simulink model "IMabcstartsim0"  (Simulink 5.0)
settings: Solver=ode45  StartTime=0.0  StopTime=4  MaxStep=1e-3  RelTol=1e-3
InitFcn:
  | imparamstartsim0
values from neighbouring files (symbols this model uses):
  Bm = 0.10    (= 0.1)    [IMabc2.m]    (also in imabcparam.m = 0.01; IMabcrun0.m = 0.01; IMabcrun1.m = 0.001; IMcur0.m = 1e-06)
  gam = 2*pi/3    (= 2.09439510239)    [IMabc2.m]    (also in IMabcf0.m; IMabcf1.m; imabcparam.m; IMabcrun0.m)
  H = 0.60    (= 0.6)    [IMabc2.m]    (also in IMcur0.m = 0.3; imdef0vec.m = 0.3; imdef1vec.m = 0.3; imdef2vec.m = 0.3)
  Lm1 = 2/3*Lm    [IMabcf0.m]    (also in IMabcf1.m; imabcparam.m = 0.0564666666667; IMabcrun0.m = 0.0564666666667; IMabcrun1.m = 0.0564666666667)
  Lr = Lrl+Lm    (= 4.6)    [IMabc2.m]    (also in IMabcf0.m = Lrl+Lm1; IMabcf1.m = Lrl+Lm1; imabcparam.m = 0.0589666666667; IMcur0.m)
  Ls = Lsl+Lm    (= 4.6)    [IMabc2.m]    (also in IMabcf0.m = Lsl+Lm1; IMabcf1.m = Lsl+Lm1; imabcparam.m = 0.0589666666667; IMcur0.m)
  Rr = input('Rotor resistance)[default = 2] =')    [Actac.m]    (also in im1phase.m = 0.3; im3d.m = eval(get(hRr,'String')); IMabc2.m = 0.02; imabcparam.m = 0.408)
  Rs = eval(get(hRs,'String'))    [im3d.m]    (also in IMabc2.m = 0.01; imabcparam.m = 0.531; IMabcrun0.m = 0.531; IMabcrun1.m = 0.531)
  Vm = Vll*sqrt(2/3)    [imabcparam.m]
  wo = 2*pi*freq0    [calc0.m]    (also in IMabc2.m = 376.991118431; imabcparam.m = 376.991118431; IMabcrun0.m = 376.991118431; IMabcrun1.m = 376.991118431)
undefined symbols (not defined in the file or in its folder): TL1, TL2
libraries: simulink x9

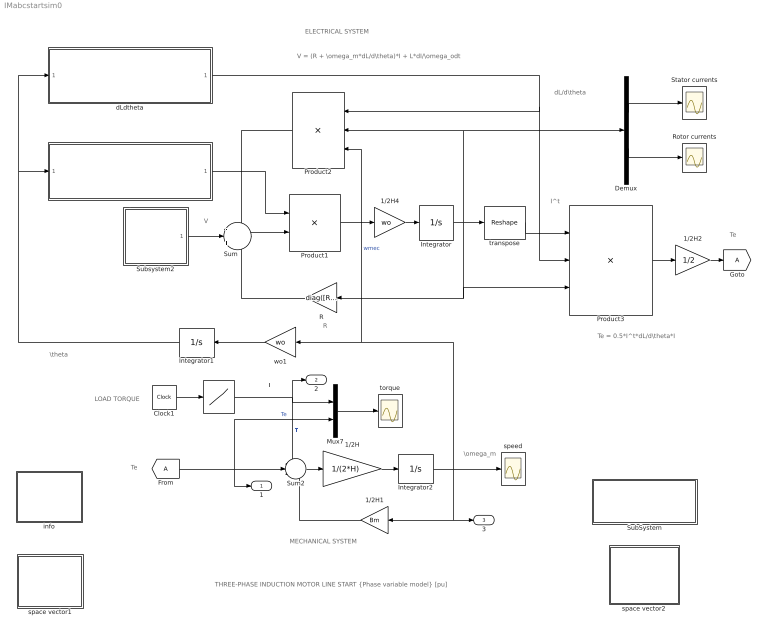
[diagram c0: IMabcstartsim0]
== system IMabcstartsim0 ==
  note: I
  note: I^t
  note: MECHANICAL SYSTEM
  note: ELECTRICAL SYSTEM
  note: V
  note: \omega_m
  note: \theta
  note: THREE-PHASE INDUCTION MOTOR LINE START {Phase variable model} [pu]
  note: L
  note: Te
  note: TL
  note: Te
  note: LOAD TORQUE
  note: R
  note: Te = 0.5*I^t*dL/d\theta*I
  note: V = (R + \omega_m*dL/d\theta)*I + L*dI/\omega_odt
  note: dL/d\theta
  " " : Lookup  InputValues="[0 2 2  4]"  OutputValues="[TL1 TL1  TL2  TL2]"
  1/2H : Gain  Gain=1/(2*H)
  1/2H1 : Gain  Orientation=left  Gain=Bm
  1/2H2 : Gain  Gain=1/2
  1/2H4 : Gain  Gain=wo
  Clock1 : Clock
  Demux : Demux  Outputs=2
  Integrator : Integrator  InitialCondition=[0 ;0 ;0; 0 ;0 ;0]
  Integrator1 : Integrator  Orientation=left
  Integrator2 : Integrator
  L : Subsystem
  Mux7 : Mux  Inputs=2
  Product1 : Product  Inputs=/*  Multiplication=Matrix(*)
  Product2 : Product  Orientation=left  Inputs=***  Multiplication=Matrix(*)
  Product3 : Product  Inputs=3  Multiplication=Matrix(*)  ShowAdditionalParam=on
  R : Gain  Orientation=left  Gain=diag([Rs Rs Rs Rr Rr Rr])  Multiplication=Matrix(K*u)
  Rotor currents : Scope
  Stator currents : Scope
  SubSystem : Subsystem
  Subsystem2 : Subsystem
  Sum : Sum  Inputs=-|+|-
  Sum2 : Sum  Inputs=-+-
  dLdtheta : Subsystem
  info : Subsystem
  space vector1 : Subsystem
  space vector2 : Subsystem
  speed : Scope
  torque : Scope
  transpose : simulink/Math Operations/Reshape  OutputDimensionality=Row vector  OutputDimensions=[1,6]
  wo1 : Gain  Orientation=left  Gain=wo
  1 : Outport
  2 : Outport  Port=2
  3 : Outport  Port=3
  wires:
  Product1/1 -> 1/2H4/1
  Sum/1 -> Product1/2
  R/1 -> Sum/3
  transpose/1 -> Product3/1
  Demux/1 -> Stator currents/1
  Demux/2 -> Rotor currents/1
  Product2/1 -> Sum/1
  dLdtheta/1(dLdtheta) -> Product2/1, Product3/2
  Product3/1 -> 1/2H2/1
  Sum2/1 -> 1/2H/1
  1/2H/1 -> Integrator2/1
  1/2H1/1 -> Sum2/3
  Mux7/1 -> torque/1
  " "/1 -> Mux7/1, Sum2/1, 2/1  "TL"
  [A] -> Sum2/2, 1/1, Mux7/2  "Te"
  Integrator2/1 -> Product2/3, wo1/1, speed/1, 1/2H1/1, 3/1  "wmec"
  Subsystem2/1(V) -> Sum/2
  Integrator1/1 -> dLdtheta/1(theta1), L/1(theta)
  L/1(L) -> Product1/1
  Clock1/1 -> " "/1
  1/2H2/1 -> [A]
  Integrator/1 -> transpose/1, Product2/2, Demux/1, R/1, Product3/3
  wo1/1 -> Integrator1/1
  1/2H4/1 -> Integrator/1

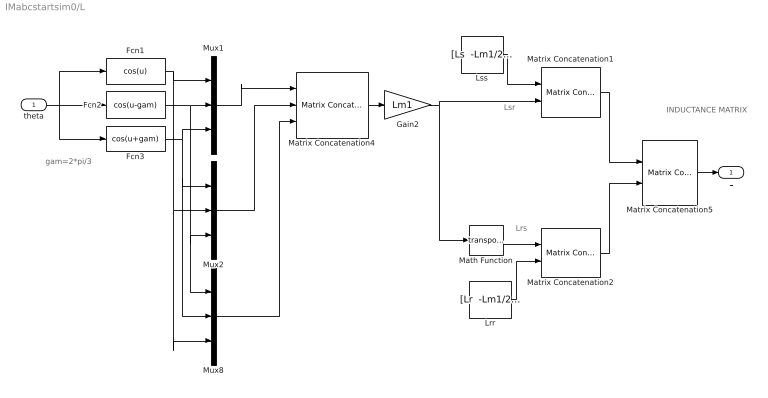
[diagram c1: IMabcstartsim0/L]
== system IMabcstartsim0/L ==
  note: Lrs
  note: Lsr
  note: INDUCTANCE MATRIX
  note: gam=2*pi/3
  theta : Inport
  Fcn1 : Fcn  Expr=cos(u)
  Fcn2 : Fcn  Expr=cos(u-gam)
  Fcn3 : Fcn  Expr=cos(u+gam)
  Gain2 : Gain  Gain=Lm1
  Lrr : Constant  Value="[Lr  -Lm1/2  -Lm1/2; -Lm1/2  Lr -Lm1/2;-Lm1/2  -Lm1/2  Lr]"  VectorParams1D=off
  Lss : Constant  Value="[Ls  -Lm1/2  -Lm1/2; -Lm1/2  Ls  -Lm1/2;-Lm1/2  -Lm1/2  Ls]"  VectorParams1D=off
  Math Function : Math  Operator=transpose
  Matrix Concatenation1 : simulink/Math Operations/Matrix Concatenation  numInports=2  catMethod=Horizontal
  Matrix Concatenation2 : simulink/Math Operations/Matrix Concatenation  numInports=2  catMethod=Horizontal
  Matrix Concatenation4 : simulink/Math Operations/Matrix Concatenation  numInports=3  catMethod=Horizontal
  Matrix Concatenation5 : simulink/Math Operations/Matrix Concatenation  numInports=2  catMethod=Vertical
  Mux1 : Mux  Inputs=3
  Mux2 : Mux  Inputs=3
  Mux8 : Mux  Inputs=3
  L : Outport
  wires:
  Fcn1/1 -> Mux1/1, Mux2/2, Mux8/3
  Fcn2/1 -> Mux8/1, Mux2/3, Mux1/2
  Fcn3/1 -> Mux8/2, Mux2/1, Mux1/3
  Lrr/1 -> Matrix Concatenation2/2
  Lss/1 -> Matrix Concatenation1/1
  Matrix Concatenation2/1 -> Matrix Concatenation5/2
  Matrix Concatenation1/1 -> Matrix Concatenation5/1
  Mux2/1 -> Matrix Concatenation4/2
  Mux8/1 -> Matrix Concatenation4/3
  Matrix Concatenation4/1 -> Gain2/1
  Mux1/1 -> Matrix Concatenation4/1
  Gain2/1 -> Math Function/1, Matrix Concatenation1/2
  Math Function/1 -> Matrix Concatenation2/1
  theta/1 -> Fcn2/1, Fcn1/1, Fcn3/1
  Matrix Concatenation5/1 -> L/1

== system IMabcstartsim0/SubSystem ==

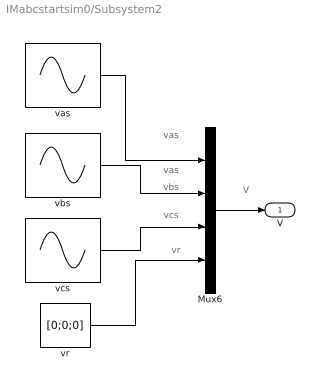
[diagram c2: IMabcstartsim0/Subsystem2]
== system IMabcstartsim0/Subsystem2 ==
  note: vas
  note: vas
  note: vbs
  note: vcs
  note: vr
  note: V
  Mux6 : Mux
  vas : Sin  Amplitude=Vm  Frequency=wo  Phase=pi/2  SampleTime=0
  vbs : Sin  Amplitude=Vm  Frequency=wo  Phase=pi/2-gam  SampleTime=0
  vcs : Sin  Amplitude=Vm  Frequency=wo  Phase=pi/2+gam  SampleTime=0
  vr : Constant  Value=[0;0;0]  VectorParams1D=off
  V : Outport
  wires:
  Mux6/1 -> V/1
  vr/1 -> Mux6/4
  vcs/1 -> Mux6/3
  vbs/1 -> Mux6/2
  vas/1 -> Mux6/1

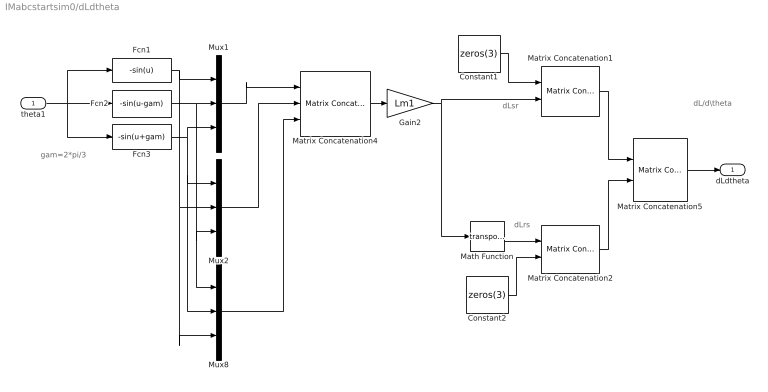
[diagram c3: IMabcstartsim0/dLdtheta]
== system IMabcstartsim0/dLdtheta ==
  note: dLrs
  note: dLsr
  note: dL/d\theta
  note: gam=2*pi/3
  theta1 : Inport
  Constant1 : Constant  Value=zeros(3)  VectorParams1D=off
  Constant2 : Constant  Value=zeros(3)  VectorParams1D=off
  Fcn1 : Fcn  Expr=-sin(u)
  Fcn2 : Fcn  Expr=-sin(u-gam)
  Fcn3 : Fcn  Expr=-sin(u+gam)
  Gain2 : Gain  Gain=Lm1
  Math Function : Math  Operator=transpose
  Matrix Concatenation1 : simulink/Math Operations/Matrix Concatenation  numInports=2  catMethod=Horizontal
  Matrix Concatenation2 : simulink/Math Operations/Matrix Concatenation  numInports=2  catMethod=Horizontal
  Matrix Concatenation4 : simulink/Math Operations/Matrix Concatenation  numInports=3  catMethod=Horizontal
  Matrix Concatenation5 : simulink/Math Operations/Matrix Concatenation  numInports=2  catMethod=Vertical
  Mux1 : Mux  Inputs=3
  Mux2 : Mux  Inputs=3
  Mux8 : Mux  Inputs=3
  dLdtheta : Outport
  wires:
  Matrix Concatenation5/1 -> dLdtheta/1
  Fcn1/1 -> Mux1/1, Mux2/2, Mux8/3
  Fcn2/1 -> Mux8/1, Mux2/3, Mux1/2
  Fcn3/1 -> Mux8/2, Mux2/1, Mux1/3
  Constant2/1 -> Matrix Concatenation2/2
  Constant1/1 -> Matrix Concatenation1/1
  Matrix Concatenation2/1 -> Matrix Concatenation5/2
  Matrix Concatenation1/1 -> Matrix Concatenation5/1
  Mux2/1 -> Matrix Concatenation4/2
  Mux8/1 -> Matrix Concatenation4/3
  Matrix Concatenation4/1 -> Gain2/1
  Mux1/1 -> Matrix Concatenation4/1
  Gain2/1 -> Math Function/1, Matrix Concatenation1/2
  Math Function/1 -> Matrix Concatenation2/1
  theta1/1 -> Fcn3/1, Fcn2/1, Fcn1/1

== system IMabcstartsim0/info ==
  note: LINE START OF AN INDUCTION MOTOR (Phase variable model) [pu]
  note: The motor is started by applying three-phase voltages to the stator. The machine dynamic equations are based on a matrix formulation using the phase variables as state variables, namely the stator currents ias, ibs, ics and the rotor currents iar, ibr, icr; the rotor speed wm; and the angular displacement between stator ax_axis and rotor ar_axis. The parameters describing the electromechanical system are expressed in per unit and may be modified by accessing a data file obtained by clicking the PARAMETERS block. The torque developed, the speed, and the stator current are observed on the scopes . The torque-speed dynamic characteristics can then be obtained after double clicking the PLOTS block. To run the identical operation of this motor now formulated in a Matlab script file, run >

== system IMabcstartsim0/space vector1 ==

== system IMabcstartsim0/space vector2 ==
